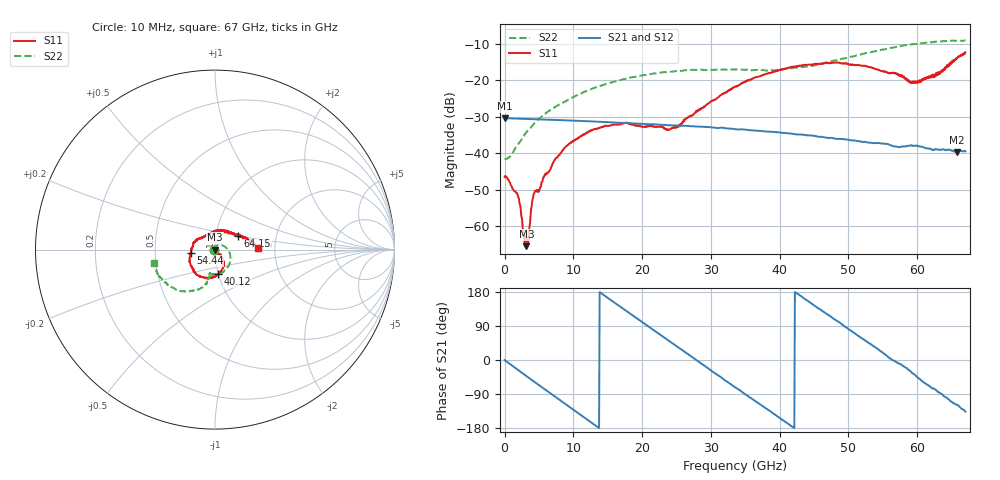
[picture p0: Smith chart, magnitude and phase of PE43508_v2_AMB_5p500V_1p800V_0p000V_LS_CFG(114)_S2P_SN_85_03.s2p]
!Keysight Technologies,N5227A,US51270237,A.10.43.00
!Date: Wednesday, August 22, 2018 17:18:35
!Correction: S11(Full 2 Port(1,3))
!S31(Full 2 Port(1,3))
!S13(Full 2 Port(1,3))
!S33(Full 2 Port(1,3))
!S2P File: Measurements: S11, S31, S13, S33:
# Hz S  dB  R 50
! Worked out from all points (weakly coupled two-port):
!   801 points, 10 MHz to 67 GHz, reference 50 ohm
!   highest |S21| = -30.43 dB at 10 MHz (marker M1); lowest = -39.7 dB at 65.74 GHz (marker M2)
!   lowest |S11| = -65.5 dB at 3.192 GHz (marker M3), VSWR 1.00, Z = 50 + j0.0479 ohm
!   |S11| at or under -10 dB: start of sweep to end of sweep
!   |S22| runs from -41.7 to -9.1 dB; largest |S21 - S12| = 0.00016
!   S11 on the Smith chart (normalised r, x): 10 MHz: 0.99, -0.00; 40.12 GHz: 1.00, -0.28; 54.44 GHz: 0.76, -0.03; 64.15 GHz: 1.27, +0.19; 67 GHz: 1.63, +0.03
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1e7  -46.56 -175.7  -30.43 -0.3  -30.43 -0.2  -41.72 -179.1
1.935962e9  -51.76 157.6  -30.56 -26.1  -30.56 -26.1  -37.60 104.9
2.857075e9  -62.95 108.1  -30.62 -38.3  -30.62 -38.3  -35.10 84.9
3.192025e9  -65.52 64.7  -30.64 -42.7  -30.65 -42.7  -34.26 79.9
3.526975e9  -63.07 10.5  -30.67 -47.1  -30.67 -47.1  -33.56 75.0
4.0294e9  -53.22 -21.6  -30.70 -53.7  -30.70 -53.7  -32.54 67.9
4.36435e9  -50.85 -12.0  -30.71 -58.0  -30.72 -58.0  -31.78 64.2
7.546375e9  -41.41 -46.4  -30.93 -99.5  -30.93 -99.5  -27.15 35.2
1.123082e10  -35.13 -65.9  -31.20 -147.3  -31.21 -147.2  -23.54 5.2
1.74274e10  -31.81 -87.8  -31.73 133.1  -31.73 133.0  -19.69 -34.4
2.236791e10  -32.73 -83.7  -32.21 69.8  -32.21 69.8  -18.06 -60.1
2.513125e10  -32.51 -65.2  -32.49 34.9  -32.48 34.8  -17.45 -71.7
3.3505e10  -21.87 -55.4  -33.43 -71.9  -33.43 -72.0  -17.08 -96.9
4.012026e10  -17.13 -82.3  -34.38 -154.5  -34.36 -154.5  -17.03 -102.0
4.472582e10  -15.72 -106.8  -35.23 147.8  -35.20 147.8  -16.08 -101.6
4.841028e10  -15.17 -126.9  -36.10 102.3  -36.10 102.3  -14.52 -103.8
5.443938e10  -17.28 -172.1  -37.29 26.8  -37.26 26.5  -11.89 -117.2
5.586291e10  -18.18 171.3  -37.66 6.3  -37.62 6.0  -11.26 -121.7
5.979858e10  -20.35 113.1  -37.95 -41.2  -37.95 -41.4  -10.12 -135.7
6.415292e10  -16.66 30.2  -39.22 -98.3  -39.26 -98.4  -9.30 -154.2
6.574394e10  -14.10 13.7  -39.69 -118.3  -39.75 -118.8  -9.19 -161.2
6.7e10  -12.37 1.8  -39.53 -136.1  -39.60 -136.1  -9.15 -167.8
